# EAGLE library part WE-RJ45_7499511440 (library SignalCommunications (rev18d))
Order Code 7499511440 Design THT xBase-T 10/100/1000 Base-T Ports 1x1 Application PoE Tab Position UP LED (Left-Right) GREEN/YELLOW-GREEN/YELLOW EMI Fingers Yes Details see: http://katalog.we-online.de/en/pbs/WE-LAN_RJ45/7499511440? Updated by Yingchun Shan 2016-08-30 2016(C) Würth Elektronik
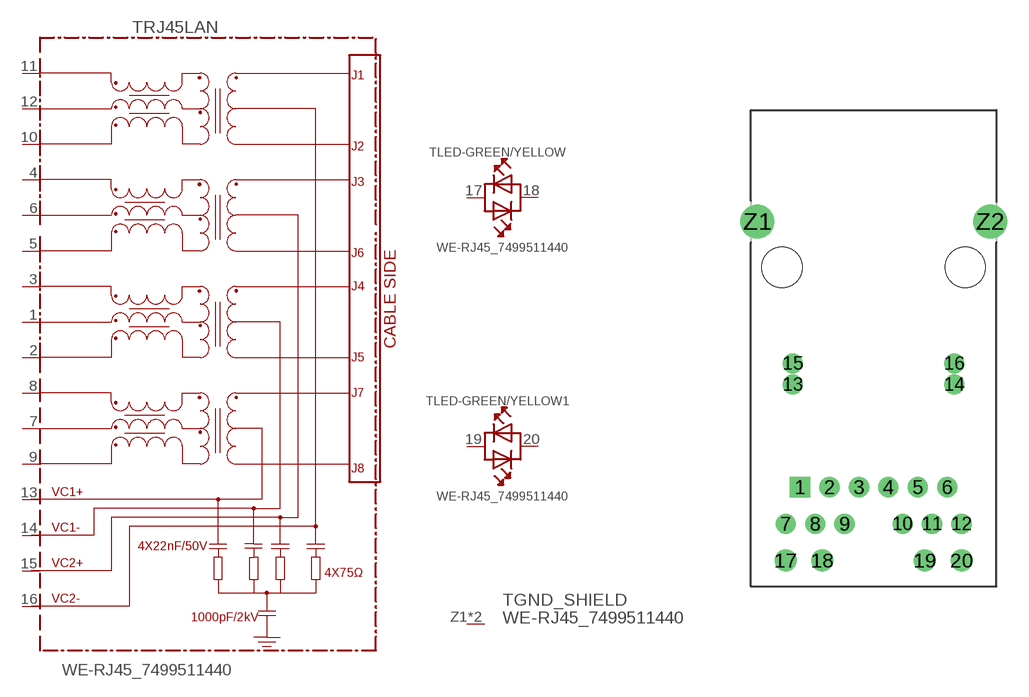
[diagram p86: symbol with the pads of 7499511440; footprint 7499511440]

Designator prefix T; gates RJ45LAN=7499511440 LED-GREEN/YELLOW=LED-DUAL-1 LED-GREEN/YELLOW1=LED-DUAL-1 GND_SHIELD=GNDPIN

## WE-RJ45_7499511440 (COMPANY-URL: http://www.we-online.de; CREATED-BY: Christin Zierenner; CREATED-DATE: AUG 2012; DATASHEET-URL: http://katalog.we-online.de/kataloge/eisos/media/pdf/7499511440.pdf; MANUFACTURER: Würth Elektronik eiSos GmbH)  [7499511440]
1  RJ45LAN:1
2  RJ45LAN:2
3  RJ45LAN:3
4  RJ45LAN:4
5  RJ45LAN:5
6  RJ45LAN:6
7  RJ45LAN:7
8  RJ45LAN:8
9  RJ45LAN:9
10  RJ45LAN:10
11  RJ45LAN:11
12  RJ45LAN:12
13  RJ45LAN:VC1+1  pwr
14  RJ45LAN:VC1-1  pwr
15  RJ45LAN:VC2+1  pwr
16  RJ45LAN:VC2-1  pwr
17  LED-GREEN/YELLOW:AK1  pas
18  LED-GREEN/YELLOW:AK2  pas
19  LED-GREEN/YELLOW1:AK1  pas
20  LED-GREEN/YELLOW1:AK2  pas
Z1  GND_SHIELD:GND  pwr
Z2  GND_SHIELD:GND  pwr

## Footprint 7499511440 (pad centres in mm)
MAX HEIGHT=13.87mm PORTS----1X1 LED -YES
drill 0.89 square: 1 -5.095,-15.24
drill 0.89: 2 -3.055,-15.24; 3 -1.015,-15.24; 4 1.015,-15.24; 5 3.055,-15.24; 6 5.095,-15.24; 7 -6.09,-17.78; 8 -4.05,-17.78; 9 -2.01,-17.78; 10 2.01,-17.78; 11 4.05,-17.78; 12 6.09,-17.78
drill 0.89 pad 1.27: 13 -5.59,-8.12; 14 5.59,-8.12; 15 -5.59,-6.66; 16 5.59,-6.66
drill 1.02: 17 -6.095,-20.32; 18 -3.555,-20.32; 19 3.555,-20.32; 20 6.095,-20.32
drill 1.57: Z1 -8.065,3.18; Z2 8.065,3.18
hole 2.8 at -6.35,0
hole 2.8 at 6.35,0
